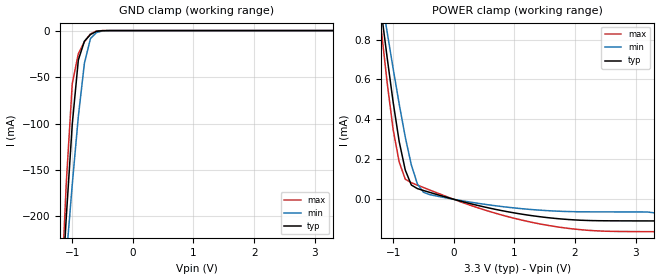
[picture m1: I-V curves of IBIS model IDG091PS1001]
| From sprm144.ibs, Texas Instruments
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[Model]   IDG091PS1001
| Input with pullup
Model_type   Input
Polarity   Non-Inverting
| signals   A, Y
Vinl = 0.8V
Vinh = 2.0V
|   typ   min   max
C_comp   1.5639p   1.4731p   1.7754p
|   typ   min   max
[Temperature Range]   25   -40   125
|   typ   min   max
[Voltage Range]   3.30V   3.00V   3.60V
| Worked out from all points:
|   GND clamp passes 1 mA (typ) near -0.61 V on its own axis
|   POWER clamp passes 1 mA (typ) near -1.22 V on its own axis
[GND_clamp]
|   Voltage   I(typ)   I(min)   I(max)
-3.3V     -2.946A    -2.225A    -3.823A
-1.2V     -314.7mA   -328.9mA   -310.5mA
-1.1V     -202mA     -245.4mA   -165.5mA
-1V       -100.6mA   -165.5mA   -57.03mA
-900mV    -31.67mA   -92.44mA   -24.94mA
-800mV    -11.48mA   -35.3mA    -12.05mA
-700mV    -4.198mA   -8.614mA   -3.556mA
-600mV    -819.1uA   -2.108mA   -409.7uA
-500mV    -75.22uA   -379.9uA   -19.35uA
-400mV    -4.217uA   -45.96uA   -434.6nA
3.3V      222pA      30.95nA    133.2pA
[POWER_clamp]
|   Voltage   I(typ)   I(min)   I(max)
-3.3V     6.292mA    5.196mA    7.209mA
-1.2V     949.4uA    1.027mA    861.9uA
-1.1V     712.2uA    838.9uA    587.3uA
-1V       486.3uA    654.6uA    348.6uA
-900mV    288.6uA    476.9uA    186.5uA
-800mV    146.5uA    311.5uA    100.8uA
-700mV    71.51uA    172uA      82.99uA
-600mV    53.57uA    76.99uA    70.93uA
-500mV    44.09uA    35.33uA    58.94uA
500mV     -38.02uA   -24.54uA   -52.48uA
1.4V      -86.44uA   -53.97uA   -122uA
3.3V      -108.3uA   -67.7uA    -162.1uA
